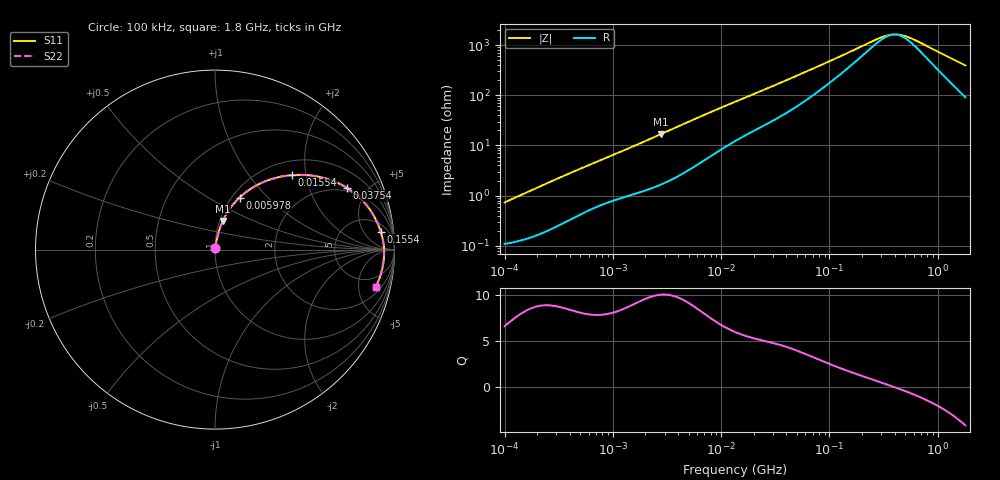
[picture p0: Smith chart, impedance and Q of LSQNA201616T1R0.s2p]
! LSQNA201616T1R0  S-PARAMETER MODEL  ( General Type )
! Model Generated by TAIYO YUDEN Corporation (http://www.ty-top.com)
! Version 2.0
! TAIYO YUDEN Control No. 100810NF25SB-FKC
! Copyright(c) 2007 TAIYO YUDEN CO.,LTD. All Rights Reserved.
! Product Description (link to TY-COMPAS)
! https://ds.yuden.co.jp/TYCOMPAS/or/detail?pn=LSQNA201616T1R0M&u=M
! Products Name : Inductors
! Characteristics :
!  Inductance : 1.0 uH , SRF(min) : 100 MHz , DC Resistance(max) : 0.117 Ohm
!  Rated Current : Saturation :600 mA , Temp Rise : 1100 mA (40 degC)
!  Case Size : 2.0 x 1.6 / 0.079 x 0.063 [mm/inch] , Thickness : 1.6 / 0.063 [mm/inch]
!  (Conditions: Temperature = 25 degC , DC Bias Current/Voltage = 0A / 0V)
! External Node Assignments :
!  1  o---GGG---o  2
! GND o---------o GND
! Frequency Range : 0.1MHz  -  1800MHz  [ 402 STEP ]
# MHz S RI R 50
! Freq[MHz].  S11 Real  S11 Imag  S21 Real  S21 Imag  S12 Real  S12 Imag  S22 Real  S22 Imag
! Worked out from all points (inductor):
!   401 points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, 100 kHz to 1.8 GHz, reference 50 ohm
!   read as one part in series: L = 1.15 uH near 105 kHz
!   highest Q = 10.1 at 2.798 MHz (marker M1), where L = 959 nH
!   self-resonance near 395.2 MHz
!   S11 on the Smith chart (normalised r, x): 100 kHz: 1.00, +0.01; 5.978 MHz: 1.08, +0.70; 15.54 MHz: 1.29, +1.67; 37.54 MHz: 1.82, +3.66; 155.4 MHz: 9, +13; 1.8 GHz: 2.83, -7.65
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0.1  0.00115 0.00725  0.9989 -0.00725  0.9989 -0.00725  0.00115 0.00725
0.516129  0.00557 0.0349  0.9944 -0.0349  0.9944 -0.0349  0.00557 0.0349
1.309209  0.0159 0.08  0.9841 -0.08  0.9841 -0.08  0.0159 0.08
2.66389  0.0398 0.152  0.9602 -0.152  0.9602 -0.152  0.0398 0.152
2.797645  0.0428 0.1588  0.9572 -0.1588  0.9572 -0.1588  0.0428 0.1588
4.242694  0.0809 0.2257  0.9191 -0.2257  0.9191 -0.2257  0.0809 0.2257
5.97828  0.1365 0.2899  0.8635 -0.2899  0.8635 -0.2899  0.1365 0.2899
8.632747  0.2276 0.3558  0.7724 -0.3558  0.7724 -0.3558  0.2276 0.3558
13.41641  0.3745 0.4078  0.6255 -0.4078  0.6255 -0.4078  0.3745 0.4078
15.54051  0.429 0.415  0.571 -0.415  0.571 -0.415  0.429 0.415
23.56755  0.5847 0.4045  0.4153 -0.4045  0.4153 -0.4045  0.5847 0.4045
37.5353  0.7363 0.343  0.2637 -0.343  0.2637 -0.343  0.7363 0.343
50.36143  0.8072 0.2879  0.1928 -0.2879  0.1928 -0.2879  0.8072 0.2879
69.24595  0.8605 0.2264  0.1395 -0.2264  0.1395 -0.2264  0.8605 0.2264
99.99243  0.8985 0.1626  0.1015 -0.1626  0.1015 -0.1626  0.8985 0.1626
155.4012  0.9235 0.1004  0.0765 -0.1004  0.0765 -0.1004  0.9235 0.1004
279.7504  0.9388 0.0346  0.0612 -0.0346  0.0612 -0.0346  0.9388 0.0346
357.3983  0.9415 0.01  0.0585 -0.01  0.0585 -0.01  0.9415 0.01
434.7684  0.9423 -0.00959  0.0577 0.00959  0.0577 0.00959  0.9423 -0.00959
542.0029  0.942 -0.0323  0.058 0.0323  0.058 0.0323  0.942 -0.0323
1024.694  0.9309 -0.1105  0.0691 0.1105  0.0691 0.1105  0.9309 -0.1105
1800  0.8954 -0.2092  0.1046 0.2092  0.1046 0.2092  0.8954 -0.2092
